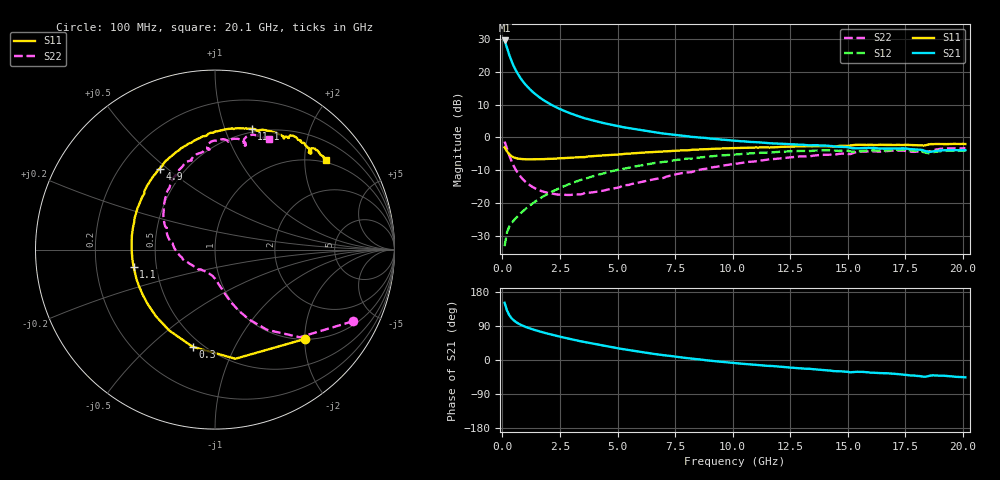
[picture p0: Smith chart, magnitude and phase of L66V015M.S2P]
!  Infineon Technologies AG
! BFR380L3 , PF131585-7, No.6, Th 09.10.01, soldered on pcb-board, measured with PP GSG850
!  Vce=6.0 V,  Ic=15.0 mA
! Common Emitter S-Parameters:  15. November 2001
#  GHz  S  MA  R  50
! f  S11  S21  S12  S22
! GHz  Mag  Ang  Mag  Ang  Mag  Ang  Mag  Ang
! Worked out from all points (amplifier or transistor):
!   201 points, 100 MHz to 20.1 GHz, reference 50 ohm
!   highest |S21| = 29.5 dB at 100 MHz (marker M1)
!   |S21| within 3 dB of that: start of sweep to 237.8 MHz
!   unconditionally stable (mu >= 1): 1.666 GHz to 4.376 GHz
!   at 3.4 GHz: K = 1.02, MAG = 8.6 dB, |S12| = -13.0 dB
!   at 10.1 GHz: K = 0.94, MSG = 2.1 dB, |S12| = -5.2 dB
!   at 20.1 GHz: K = 0.99, MSG = 0.1 dB, |S12| = -4.0 dB
!   S11 on the Smith chart (normalised r, x): 100 MHz: 1.01, -1.99; 300 MHz: 0.44, -0.70; 1.1 GHz: 0.37, -0.09; 4.9 GHz: 0.37, +0.47; 11.1 GHz: 0.47, +1.24; 20.1 GHz: 0.94, +2.52
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0.1  0.7053 -45.0  29.88 151.0  0.02213 67.5  0.8656 -27.5
0.2  0.6186 -79.5  23.24 131.1  0.03568 57.8  0.6794 -45.9
0.3  0.5557 -102.9  18.11 118.7  0.04365 53.5  0.5335 -57.0
0.4  0.5178 -119.5  14.57 110.4  0.04979 52.1  0.4338 -64.0
0.5  0.4965 -131.4  12.07 104.5  0.05455 52.8  0.3645 -68.8
0.6  0.4826 -140.9  10.28 99.9  0.05982 53.5  0.3154 -72.3
0.7  0.4748 -148.2  8.949 96.1  0.06494 54.5  0.2788 -75.1
0.8  0.4697 -154.4  7.9 92.9  0.07037 55.7  0.2512 -77.4
0.9  0.4673 -159.5  7.072 90.2  0.07557 56.7  0.2291 -79.4
1.1  0.4632 -168.0  5.859 85.4  0.08698 58.3  0.1985 -83.2
1.3  0.4634 -174.7  4.998 81.2  0.09802 59.5  0.1773 -86.5
1.5  0.4647 179.3  4.365 77.4  0.1098 60.2  0.1628 -89.8
2  0.4705 167.8  3.325 69.0  0.1397 60.5  0.1427 -98.6
2.6  0.4825 156.5  2.61 60.2  0.1761 59.3  0.1341 -110.5
3.5  0.5016 142.3  1.995 48.3  0.2313 55.6  0.1384 -127.2
4.9  0.546 124.5  1.515 32.2  0.314 48.1  0.1687 -155.9
6.8  0.6058 104.6  1.173 14.2  0.4173 35.9  0.2372 172.6
10.1  0.6883 79.4  0.8886 -8.0  0.5509 14.5  0.3967 134.4
11.1  0.7008 73.1  0.843 -13.3  0.5804 7.9  0.4389 124.6
13.5  0.7342 61.3  0.7597 -24.1  0.627 -6.9  0.5263 103.9
16.8  0.7698 48.6  0.6794 -35.3  0.6362 -23.5  0.6238 81.0
20.1  0.7926 39.0  0.6402 -45.8  0.6291 -37.5  0.6842 64.0
